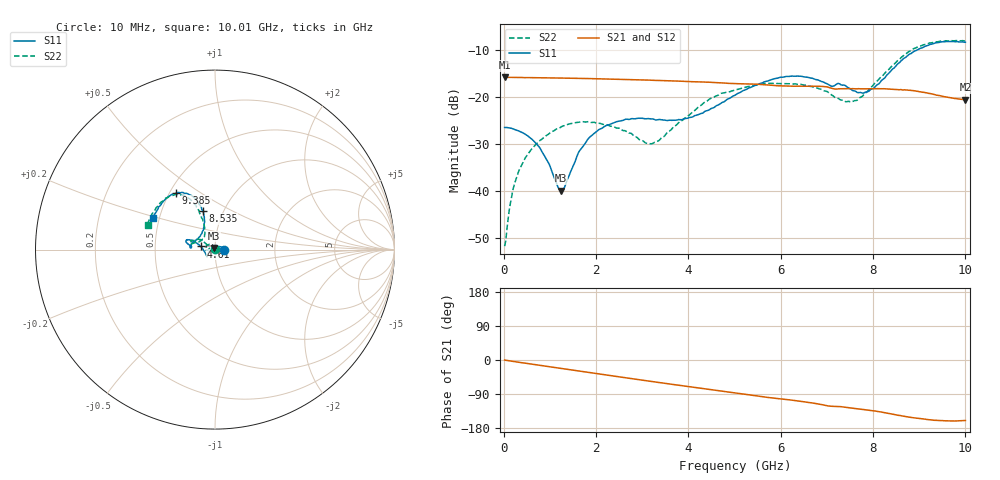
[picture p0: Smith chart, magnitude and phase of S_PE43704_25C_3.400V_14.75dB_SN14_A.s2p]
! Device ID: PE43704
! Dir: z:\PE43704\PE43704_Char_1_20130516\PE43704\AMB\3p400V\14p75dB
! Serial: 14
! Insertion: A
! Impedance: 50 ohm
! Temp: Amb
! VDD: 3.400V
! Attenuation Step: 14.75dB
! IDD: 1.139268e-01mA
#  Hz  S  RI  R  50
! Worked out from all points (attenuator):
!   401 points, 10 MHz to 10.01 GHz, reference 50 ohm
!   highest |S21| = -15.72 dB at 10 MHz (marker M1); lowest = -20.5 dB at 10.01 GHz (marker M2)
!   lowest |S11| = -39.8 dB at 1.235 GHz (marker M3), VSWR 1.02, Z = 49.6 + j0.921 ohm
!   |S11| at or under -10 dB: start of sweep to 8.944 GHz
!   |S22| runs from -51.7 to -7.9 dB; largest |S21 - S12| = 0.0016
!   S11 on the Smith chart (normalised r, x): 10 MHz: 1.10, +0.00; 4.61 GHz: 0.85, +0.03; 8.535 GHz: 0.80, +0.36; 9.385 GHz: 0.54, +0.40; 10.01 GHz: 0.46, +0.19
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1e7  0.0479 0.000154  0.1637 -0.000565  0.1638 -0.000584  -0.00255 0.000565
1.85e8  0.0461 0.0057  0.163 -0.00985  0.163 -0.00984  -0.00276 0.00976
3.85e8  0.0411 0.0111  0.1617 -0.0205  0.1613 -0.0204  -0.00637 0.0181
7.6e8  0.0242 0.0172  0.1572 -0.0387  0.1573 -0.0386  -0.0196 0.0282
1.235e9  -0.00418 0.00929  0.1487 -0.0609  0.1488 -0.0608  -0.0411 0.0258
1.685e9  -0.0276 -0.00822  0.1377 -0.0801  0.1378 -0.08  -0.054 0.0119
2.01e9  -0.0381 -0.0213  0.1281 -0.0928  0.128 -0.0925  -0.053 0.00219
2.41e9  -0.0429 -0.0336  0.1145 -0.1066  0.1146 -0.1065  -0.0479 -0.00349
3.11e9  -0.0456 -0.0384  0.0876 -0.1255  0.0878 -0.1254  -0.0319 0.00572
3.36e9  -0.0476 -0.0336  0.0771 -0.1304  0.0773 -0.1302  -0.032 0.0136
4.035e9  -0.0608 -0.00824  0.0485 -0.1391  0.0485 -0.1393  -0.0551 0.0367
4.61e9  -0.08 0.0174  0.0234 -0.1418  0.0238 -0.1417  -0.0873 0.0569
5.01e9  -0.0998 0.0346  0.00775 -0.1402  0.00772 -0.1404  -0.1075 0.0525
5.96e9  -0.1521 0.0552  -0.0278 -0.13  -0.0274 -0.1299  -0.1345 0.0406
6.685e9  -0.1562 0.0354  -0.0524 -0.1206  -0.0522 -0.1207  -0.1258 0.0337
7.585e9  -0.1042 0.0545  -0.0755 -0.0981  -0.0755 -0.0979  -0.0628 0.0669
7.91e9  -0.0733 0.0898  -0.0833 -0.0911  -0.0833 -0.0916  -0.0556 0.1063
8.36e9  -0.0596 0.1734  -0.0957 -0.0767  -0.0957 -0.0769  -0.0763 0.1864
8.535e9  -0.0696 0.2154  -0.0997 -0.0689  -0.0992 -0.07  -0.0966 0.2257
8.935e9  -0.1181 0.2917  -0.1045 -0.0529  -0.1041 -0.0519  -0.1625 0.2951
9.385e9  -0.2158 0.3151  -0.0988 -0.0375  -0.0993 -0.0371  -0.2584 0.2933
1.001e10  -0.3453 0.1742  -0.0888 -0.033  -0.0902 -0.0329  -0.3758 0.1361
